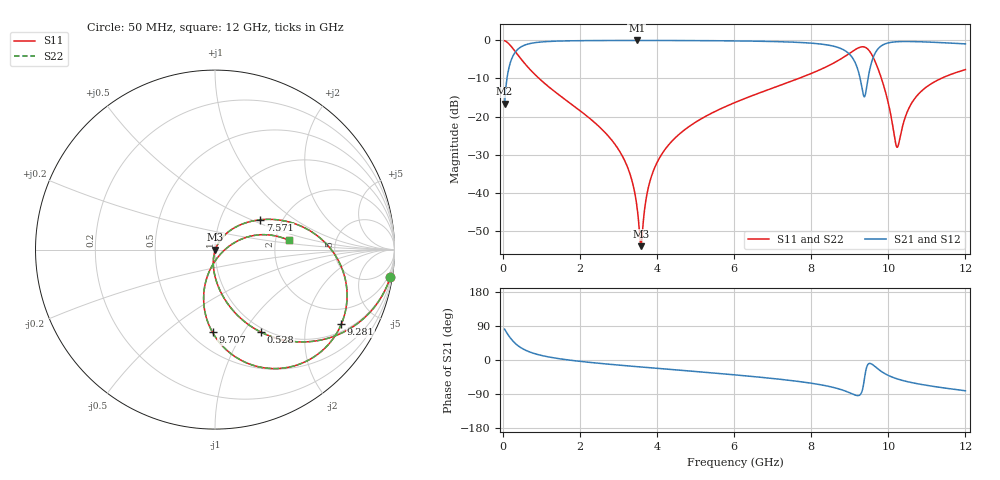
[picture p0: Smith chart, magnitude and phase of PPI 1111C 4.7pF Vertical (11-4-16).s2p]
# GHz S MA R 50
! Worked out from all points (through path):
!   1601 points, 50 MHz to 12 GHz, reference 50 ohm
!   highest |S21| = -0.02 dB at 3.478 GHz (marker M1); lowest = -16.6 dB at 50 MHz (marker M2)
!   group delay of S21, straight-line fit = 23 ps
!   lowest |S11| = -54.1 dB at 3.583 GHz (marker M3), VSWR 1.00, Z = 50.2 - j0.0792 ohm
!   |S11| at or under -10 dB: 944.2 MHz to 7.676 GHz (6.732 GHz wide, 156 % of centre); 9.823 GHz to 11.37 GHz (1.547 GHz wide, 14.6 % of centre)
!   |S22| runs from -54.1 to -0.1 dB; largest |S21 - S12| = 0
!   S11 on the Smith chart (normalised r, x): 50 MHz: 1, -13; 528 MHz: 0.94, -1.21; 7.571 GHz: 1.55, +0.57; 9.281 GHz: 1.28, -3.19; 9.707 GHz: 0.63, -0.74; 12 GHz: 2.36, +0.30
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0.05  0.989 -8.8  0.1477 81.2  0.1477 81.2  0.989 -8.8
0.22925  0.8241 -35.7  0.566 54.3  0.566 54.3  0.8241 -35.7
0.528  0.5283 -60.8  0.8483 29.1  0.8483 29.1  0.5283 -60.8
2.044156  0.1153 -93.3  0.9918 -4.0  0.9918 -4.0  0.1153 -93.3
3.059906  0.03316 -100.8  0.9975 -13.9  0.9975 -13.9  0.03316 -100.8
3.321312  0.01636 -99.6  0.9978 -16.2  0.9978 -16.2  0.01636 -99.6
3.478156  0.006815 -91.0  0.9978 -17.5  0.9978 -17.5  0.006815 -91.0
3.582719  0.001983 -23.4  0.9978 -18.4  0.9978 -18.4  0.001983 -23.4
3.784375  0.01207 60.1  0.9977 -20.1  0.9977 -20.1  0.01207 60.1
4.038312  0.02693 63.2  0.9973 -22.3  0.9973 -22.3  0.02693 63.2
4.747844  0.06873 59.8  0.9949 -28.2  0.9949 -28.2  0.06873 59.8
6.025  0.1528 49.5  0.9846 -39.3  0.9846 -39.3  0.1528 49.5
7.571031  0.302 33.4  0.9462 -55.3  0.9462 -55.3  0.302 33.4
8.019156  0.3705 26.9  0.9182 -61.5  0.9182 -61.5  0.3705 26.9
8.848187  0.6041 4.8  0.7483 -80.5  0.7483 -80.5  0.6041 4.8
9.281375  0.8172 -30.6  0.2964 -90.4  0.2964 -90.4  0.8172 -30.6
9.393406  0.8143 -46.8  0.1858 -41.7  0.1858 -41.7  0.8143 -46.8
9.707094  0.4613 -91.7  0.7441 -21.5  0.7441 -21.5  0.4613 -91.7
10.01331  0.1404 -105.5  0.9304 -41.3  0.9304 -41.3  0.1404 -105.5
10.23738  0.03957 -37.2  0.9608 -50.0  0.9608 -50.0  0.03957 -37.2
10.77512  0.1952 21.2  0.9607 -63.0  0.9607 -63.0  0.1952 21.2
12  0.413 7.3  0.8992 -81.2  0.8992 -81.2  0.413 7.3
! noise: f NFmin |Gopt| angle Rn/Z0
0.05  0.0004712  0.9056  2.422  0.001095
1.372  0.004023  0.693  7.964  0.002542
2.701  0.006611  0.6454  14.3  0.003479
4.031  0.009082  0.6252  20.52  0.004398
5.36  0.01184  0.6256  26.56  0.005624
6.682  0.01591  0.6554  32.49  0.008142
8.012  0.02752  0.7544  38.82  0.02019
9.341  0.4987  0.9827  45.65  5.591
10.67  0.04369  0.8018  51.1  0.03733
12  0.03367  0.7334  55.49  0.01987
